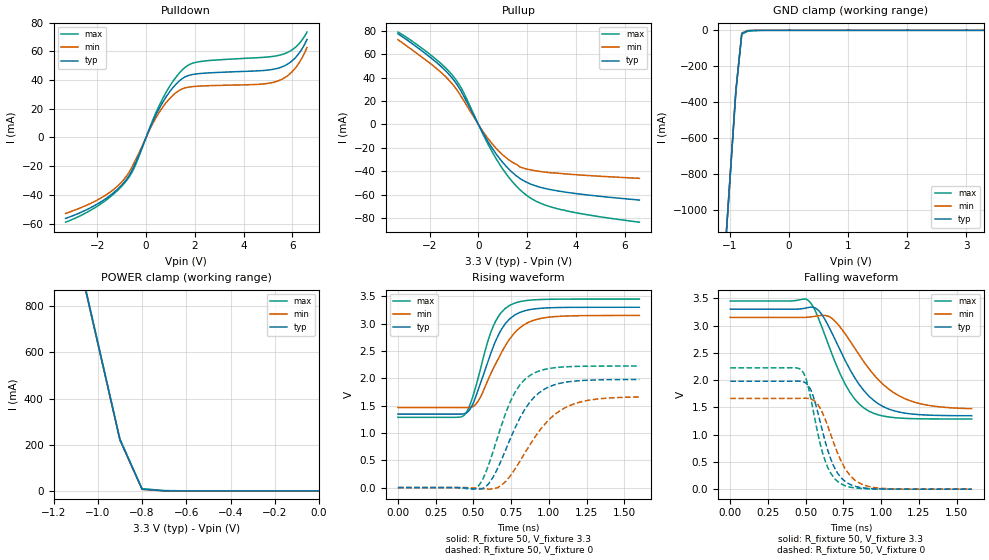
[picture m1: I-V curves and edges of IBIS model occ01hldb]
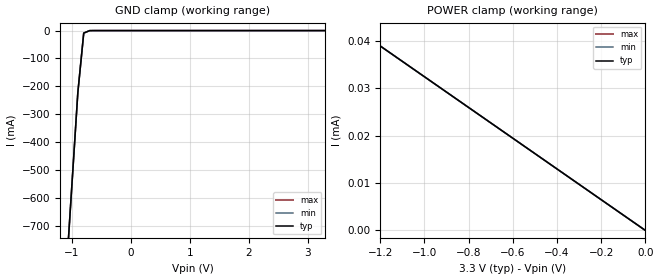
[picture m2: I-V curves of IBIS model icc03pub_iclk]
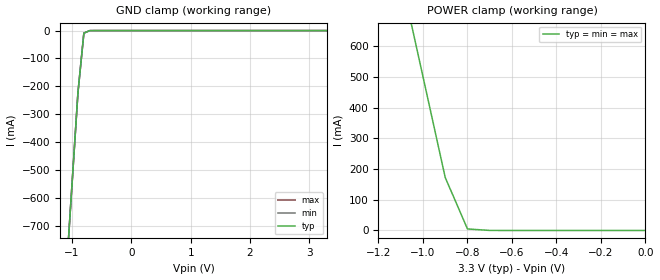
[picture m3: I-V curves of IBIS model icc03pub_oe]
|   MPC94551   I B I S   M O D E L   |
|   F R E E S C A L E   S E M I C O N D U C T O R   |
[IBIS Ver]   3.2
[File name]   mpc94551.ibs
[File Rev]   1.0
[Date]   30-Mar-05 12:58:12 PM
[Source]   This file was generated from transistor-level
|   simulations
[Notes]
[Disclaimer]   This information is for modeling purposes only,
|   and is not guaranteed.
[Copyright]   Copyright 2005, Freescale Semiconductor.,
|   All Rights Reserved.
|   MPC94551
|   8-PIN SOIC PACKAGE
|   C O M P O N E N T  D E S C R I P T I O N
[Component]   mpc94551
[Manufacturer]   Freescale Semiconductor, Inc.
[Package]
R_pkg   46.8m   25.9m   59.1m
L_pkg   2.18nH   1.14nH   2.67nH
C_pkg   0.128pF   0.0891pF   0.160pF
[Pin] signal_name   model_name   R_pin   L_pin   C_pin
1   ICLK   icc03pub_iclk   59.1m   2.67nH   0.122pF
2   Q1   occ01hldb   51.9m   2.29nH   0.0891pF
3   Q2   occ01hldb   54.3m   2.37nH   0.115pF
4   Q3   occ01hldb   29.8m   1.46nH   0.160pF
5   Q4   occ01hldb   42.6m   2.49nH   0.140pF
6   GND   GND   25.9m   1.14nH   0.124pF
7   VDD   POWER   51.5m   2.32nH   0.110pF
8   OE   icc03pub_oe   59.1m   2.67nH   0.160pF
| Models and submodels in the file (3): occ01hldb (3-state), icc03pub_iclk (Input), icc03pub_oe (Input)
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|   M O D E L  S T A T E M E N T
[Model]   occ01hldb
Model_type   3-state
Enable   Active-Low
Polarity   Non-Inverting
Vref   =  1.65
Vmeas   =  1.65
Rref   =  50
Cref   =  15pF
C_comp   4pF   4pF   4pF
[Temperature Range] 55   110   0
[Voltage Range]   3.3   3.15   3.45
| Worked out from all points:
|   slope of the pulldown table from 0 to 0.495 V, typ, clamps not added: 26.4 ohm
|   slope of the pullup table from 0 to 0.495 V, typ, clamps not added: 27.5 ohm
|   GND clamp passes 1 mA (typ) near -0.62 V on its own axis
|   POWER clamp passes 1 mA (typ) near -0.71 V on its own axis
|   falling waveform, R_fixture 50, V_fixture 3.3: 20-80 % time 243ps typ, 292ps min, 207ps max; typ from 3.3 V to 1.35 V
|   falling waveform, R_fixture 50, V_fixture 0: 20-80 % time 128ps typ, 150ps min, 115ps max; typ from 1.98 V to 0 V
|   rising waveform, R_fixture 50, V_fixture 3.3: 20-80 % time 165ps typ, 196ps min, 140ps max; typ from 1.34 V to 3.3 V
|   rising waveform, R_fixture 50, V_fixture 0: 20-80 % time 212ps typ, 261ps min, 180ps max; typ from 0 V to 1.98 V
[Pullup]
-3.3V     77.37mA    72.3mA     78.82mA
-1.9V     56.03mA    50.84mA    58.37mA
-1.4V     46.92mA    41.89mA    49.37mA
-1V       37.61mA    32.79mA    40.27mA
-600mV    24.15mA    20.3mA     27.06mA
200mV     -7.722mA   -6.378mA   -8.83mA
700mV     -24.33mA   -19.74mA   -28.25mA
1.3V      -39.16mA   -30.89mA   -46.49mA
1.9V      -48.48mA   -37.54mA   -59.2mA
2.5V      -53.33mA   -39.98mA   -66.76mA
3.3V      -56.85mA   -41.66mA   -72.19mA
6.6V      -64.46mA   -45.92mA   -83.35mA
[Pulldown]
-3.3V     -56.4mA    -52.99mA   -59.04mA
-1.7V     -43.17mA   -40.64mA   -44.42mA
-800mV    -29.18mA   -26.95mA   -30.03mA
-500mV    -20.29mA   -18.04mA   -21.74mA
200mV     8.214mA    7.199mA    8.969mA
600mV     22.02mA    19.04mA    24.33mA
1.1V      34.69mA    29.35mA    39.03mA
1.6V      42.18mA    34.5mA     48.81mA
2.3V      44.64mA    35.85mA    53.05mA
5.4V      48.18mA    39.29mA    57.03mA
6.1V      55.14mA    47.86mA    62.44mA
6.6V      68.22mA    62.62mA    73.39mA
[GND Clamp]
-3.3V     -12.05A    -12.03A    -12.06A
-1.1V     -1.31A     -1.305A    -1.316A
-1V       -822.3mA   -818.1mA   -827.3mA
-900mV    -334.7mA   -331.3mA   -339.1mA
-800mV    -17.61mA   -15.09mA   -21.26mA
-700mV    -2.45mA    -936.3uA   -5.219mA
-400mV    -10.9uA    -868.7nA   -101.1uA
3.3V      101.6pA    13.62pA    5.428nA
[POWER Clamp]
-3.3V     10.34A     10.31A     10.37A
-1.1V     1.059A     1.055A     1.065A
-1V       640.2mA    637.4mA    644.7mA
-900mV    221.6mA    219.7mA    225mA
-800mV    7.523mA    6.588mA    9.847mA
-700mV    438.3uA    172.2uA    1.616mA
-600mV    46.56uA    6.55uA     380.7uA
0V        101.6pA    7.972pA    6.308nA
[Falling Waveform]
R_fixture=50
V_fixture=3.3
V_fixture_min=3.15
V_fixture_max=3.45
0s        3.3V       3.15V      3.45V
517.2ps   3.33V      3.154V     3.461V
581.8ps   3.286V     3.178V     3.151V
678.8ps   2.837V     3.12V      2.444V
791.9ps   2.201V     2.725V     1.781V
921.2ps   1.701V     2.202V     1.428V
1.051ns   1.469V     1.835V     1.324V
1.18ns    1.386V     1.634V     1.296V
1.341ns   1.355V     1.525V     1.288V
1.6ns     1.346V     1.476V     1.286V
[Falling Waveform]
R_fixture=50
V_fixture=0
V_fixture_min=0
V_fixture_max=0
0s        1.979V     1.664V     2.225V
468.7ps   1.978V     1.666V     2.191V
501ps     1.947V     1.668V     2.037V
533.3ps   1.822V     1.655V     1.672V
598ps     1.208V     1.476V     806.3mV
630.3ps   861.7mV    1.274V     506.7mV
727.3ps   235.9mV    557mV      107.9mV
824.2ps   55.72mV    169.5mV    22.49mV
921.2ps   13.22mV    46.96mV    4.905mV
1.6ns     2.408uV    20.62uV    488.8nV
[Rising Waveform]
R_fixture=50
V_fixture=3.3
V_fixture_min=3.15
V_fixture_max=3.45
0s        1.345V     1.465V     1.286V
436.4ps   1.35V      1.464V     1.317V
468.7ps   1.4V       1.466V     1.455V
517.2ps   1.675V     1.527V     1.859V
630.3ps   2.565V     2.169V     2.943V
678.8ps   2.863V     2.431V     3.184V
743.4ps   3.094V     2.729V     3.339V
824.2ps   3.221V     2.959V     3.411V
953.5ps   3.283V     3.099V     3.442V
1.6ns     3.3V       3.15V      3.45V
[Rising Waveform]
R_fixture=50
V_fixture=0
V_fixture_min=0
V_fixture_max=0
0s        461.5pV    111pV      39.75nV
533.3ps   -28.29mV   -13.43mV   29.84mV
565.7ps   -10.03mV   -22.3mV    171.9mV
630.3ps   191.1mV    -23.38mV   658.1mV
759.6ps   987.3mV    273.3mV    1.657V
824.2ps   1.352V     555.5mV    1.929V
905.1ps   1.661V     912.8mV    2.099V
1.018ns   1.862V     1.286V     2.186V
1.147ns   1.942V     1.511V     2.215V
1.6ns     1.978V     1.658V     2.225V
[Ramp]
R_load=50
dV/dt_r   1.187E+0/2.122E-10   9.950E-1/2.606E-10   1.335E+0/1.794E-10
dV/dt_f   1.172E+0/2.430E-10   1.004E+0/2.922E-10   1.298E+0/2.066E-10
|[End   occ01hldb
|   icc03pub_iclk   INPUT MODEL WITH A 31K PULLUP RESISTOR
[Model]   icc03pub_iclk
Model_type  Input
Vinh   =  2.1
Vinl   =  1.1
C_comp   5pF   5pF   5pF
[Temperature Range] 55   110   0
[Voltage Range]   3.3   3.15   3.45
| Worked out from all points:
|   GND clamp passes 1 mA (typ) near -0.71 V on its own axis
|   POWER clamp passes 1 mA (typ) near -2.25 V on its own axis
[GND Clamp]
-3.3V     -8.11A     -8.11A     -8.11A
-1.1V     -879.4mA   -879.4mA   -879.4mA
-1V       -550.8mA   -550.8mA   -550.8mA
-900mV    -222.2mA   -222.2mA   -222.2mA
-800mV    -8.936mA   -8.936mA   -8.936mA
-700mV    -187.1uA   -187.1uA   -187.1uA
3.3V      5.288nA    5.288nA    5.288nA
[POWER Clamp]
-3.3V     830.1mA    830.1mA    830.1mA
-1.3V     42.14uA    42.14uA    42.14uA
-1V       32.42uA    32.42uA    32.42uA
0V        5.288nA    4.992nA    5.583nA
|   icc03pub_oe   INPUT MODEL WITH A 31K PULLUP RESISTOR
[Model]   icc03pub_oe
Model_type  Input
Vinh   =  2.0
Vinl   =  0.8
C_comp   5pF   5pF   5pF
[Temperature Range] 55   110   0
[Voltage Range]   3.3   3.15   3.45
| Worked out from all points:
|   GND clamp passes 1 mA (typ) near -0.71 V on its own axis
|   POWER clamp passes 1 mA (typ) near -0.72 V on its own axis
[GND Clamp]
-3.3V     -8.11A     -8.11A     -8.11A
-1.1V     -879.4mA   -879.4mA   -879.4mA
-1V       -550.8mA   -550.8mA   -550.8mA
-900mV    -222.2mA   -222.2mA   -222.2mA
-800mV    -8.936mA   -8.936mA   -8.936mA
-700mV    -187.1uA   -187.1uA   -187.1uA
3.3V      0A         2.323pA    0A
[POWER Clamp]
-3.3V     8.06A      8.06A      8.06A
-1.1V     830mA      830mA      830mA
-1V       501.3mA    501.3mA    501.3mA
-900mV    172.7mA    172.7mA    172.7mA
-800mV    5.017mA    5.017mA    5.017mA
-700mV    127.2uA    127.2uA    127.2uA
0V        0A         0A         0A
